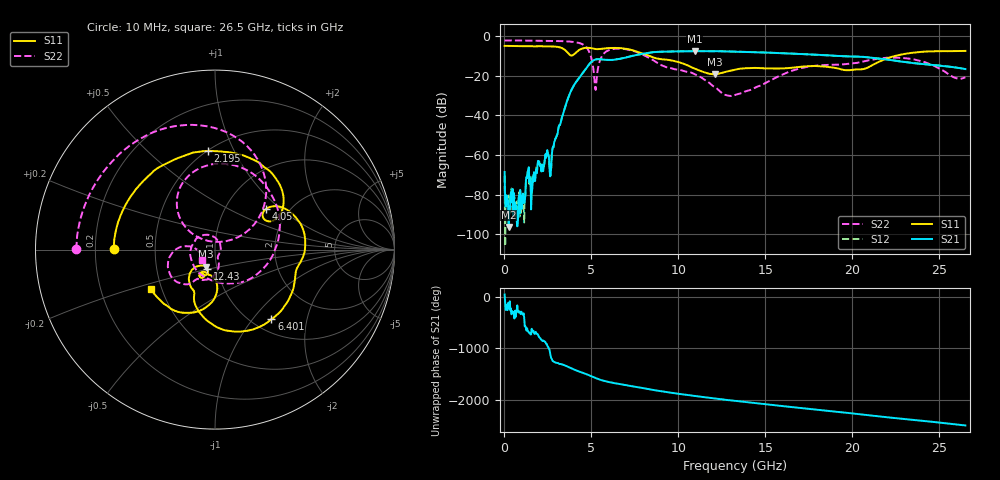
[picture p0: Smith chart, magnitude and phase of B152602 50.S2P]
!  2-Port S-parameters saved by WinCal
! VAR MeasName=S-Parameters (CALIBRATED_DATA) read from VNA (N5242A)
! VAR MeasDate=2016-1-5 16:33:15
! VAR NAME=B152602 50
! VAR FILENAME=B152602 50.S2P
! VAR DATE=2016-1-5 16:33:15
! VAR PHYS_PORTS=1,2
# Hz S DB R 50
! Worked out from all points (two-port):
!   801 points, 10 MHz to 26.5 GHz, reference 50 ohm
!   highest |S21| = -7.62 dB at 10.94 GHz (marker M1); lowest = -96.2 dB at 241.8 MHz (marker M2)
!   |S21| within 3 dB of the highest: 7.078 GHz to 20.74 GHz (13.67 GHz wide, 98.2 % of centre)
!   lowest |S11| = -19.4 dB at 12.1 GHz (marker M3), VSWR 1.24, Z = 44.3 - j8.45 ohm
!   |S11| at or under -10 dB: 8.32 GHz to 22.48 GHz (14.16 GHz wide, 91.9 % of centre)
!   |S22| runs from -30.3 to -2.2 dB; largest |S21 - S12| = 0.0033
!   S11 on the Smith chart (normalised r, x): 10 MHz: 0.28, +0.00; 2.195 GHz: 0.50, +0.79; 4.05 GHz: 1.54, +0.80; 6.401 GHz: 1.21, -1.25; 12.43 GHz: 0.90, -0.20; 26.5 GHz: 0.43, -0.23
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1e7  -4.98 179.5  -68.52 51.8  -70.37 131.5  -2.25 179.8
2.417875e8  -4.99 170.5  -96.22 -166.3  -90.89 -88.4  -2.25 176.3
1.0696e9  -5.14 139.0  -79.44 18.6  -79.55 63.7  -2.30 163.4
1.367612e9  -5.10 127.6  -67.46 51.8  -71.39 55.8  -2.33 158.7
2.195425e9  -5.18 94.2  -67.48 -135.4  -67.18 -138.0  -2.41 144.8
2.692112e9  -5.23 72.7  -64.43 -110.4  -66.42 -106.3  -2.46 135.3
4.049725e9  -8.81 38.6  -24.05 22.0  -24.07 22.0  -3.09 98.0
4.447075e9  -6.42 23.9  -19.30 -29.6  -19.28 -29.5  -3.98 78.5
4.877538e9  -5.99 1.3  -14.19 -84.3  -14.19 -84.1  -8.05 44.7
5.241775e9  -6.57 -12.2  -11.81 -137.6  -11.80 -137.5  -27.16 98.3
5.672238e9  -6.34 -23.9  -11.88 172.1  -11.87 172.3  -9.30 128.4
6.400712e9  -6.04 -51.0  -11.87 118.4  -11.85 118.6  -6.40 88.1
7.625875e9  -7.87 -95.0  -9.50 44.6  -9.46 44.6  -8.20 21.9
8.851038e9  -11.47 -115.6  -7.97 -26.7  -7.94 -26.8  -13.92 -69.7
1.093712e10  -16.43 -138.3  -7.62 -127.4  -7.63 -127.4  -19.23 135.1
1.209606e10  -19.37 -118.8  -7.66 -176.2  -7.67 -176.2  -25.65 68.8
1.242719e10  -18.75 -111.5  -7.70 169.8  -7.67 169.9  -28.15 40.4
1.3255e10  -17.00 -107.4  -7.87 137.1  -7.85 137.0  -29.77 -40.0
1.504308e10  -16.35 -115.9  -8.34 69.6  -8.35 69.4  -23.51 -73.7
1.769208e10  -15.12 -116.3  -9.32 -26.4  -9.30 -26.2  -15.20 -106.1
2.209604e10  -10.95 -92.0  -12.01 173.6  -11.93 173.6  -10.92 -145.1
2.65e10  -7.51 -148.4  -16.67 17.2  -16.66 17.0  -20.77 -142.4
